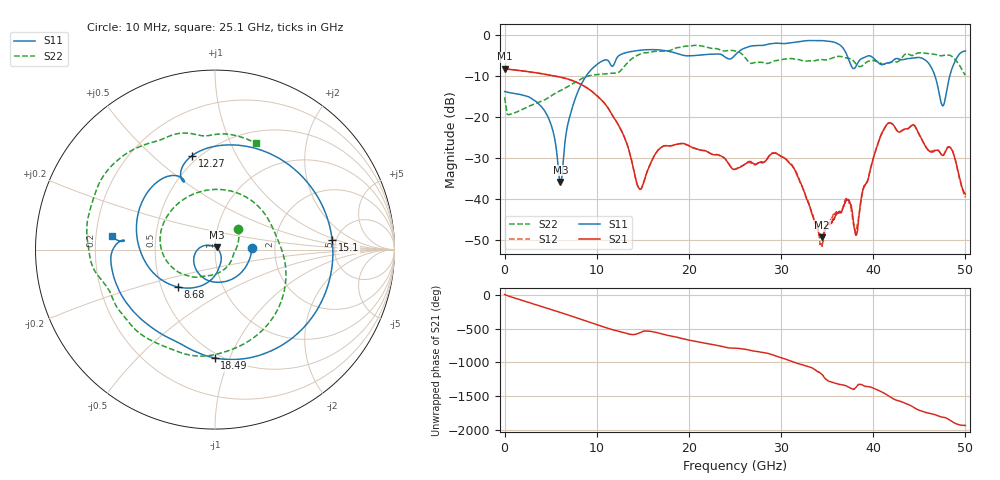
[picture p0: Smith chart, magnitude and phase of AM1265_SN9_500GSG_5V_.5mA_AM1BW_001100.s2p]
!Keysight Technologies,N5245B,MY58422270,A.16.20.02
!Date: Thursday, March 05, 2026 00:39:02
!Correction: S11(C  2-Port  )
!S21(C  2-Port  )
!S12(C  2-Port  )
!S22(C  2-Port  )
!S2P File: Measurements: S11, S21, S12, S22:
# Hz S  dB  R 50
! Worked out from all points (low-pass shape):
!   3201 points, 10 MHz to 50 GHz, reference 50 ohm
!   highest |S21| = -8.27 dB at 10 MHz (marker M1); lowest = -49.3 dB at 34.44 GHz (marker M2)
!   |S21| within 3 dB of the highest: start of sweep to 7.521 GHz
!   lowest |S11| = -35.8 dB at 6.071 GHz (marker M3), VSWR 1.03, Z = 50.9 + j1.37 ohm
!   |S11| at or under -10 dB: start of sweep to 8.867 GHz; 46.7 GHz to 48.3 GHz (1.608 GHz wide, 3.39 % of centre)
!   |S22| runs from -19.4 to -2.6 dB; largest |S21 - S12| = 0.0041
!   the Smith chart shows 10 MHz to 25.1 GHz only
!   S11 on the Smith chart (normalised r, x): 10 MHz: 1.51, +0.02; 8.68 GHz: 0.61, -0.28; 12.27 GHz: 0.46, +0.68; 15.1 GHz: 4.64, +0.85; 18.49 GHz: 0.46, -0.88; 25.1 GHz: 0.27, +0.06
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1e7  -13.80 2.2  -8.27 3.7  -8.33 3.3  -15.22 41.6
2.072088e9  -14.73 -83.3  -8.81 -88.3  -8.81 -88.3  -18.01 -72.4
4.337259e9  -18.48 -164.4  -9.58 175.5  -9.58 175.5  -15.85 -113.1
6.071288e9  -35.84 56.5  -10.30 99.6  -10.30 99.6  -13.57 -135.9
8.352081e9  -11.95 -122.1  -12.13 -5.1  -12.12 -5.0  -10.69 -175.6
8.680141e9  -10.65 -134.8  -12.55 -20.3  -12.53 -20.2  -10.35 176.2
1.227317e10  -5.37 103.7  -21.62 -177.0  -21.61 -176.8  -9.24 17.7
1.510073e10  -3.67 4.6  -35.94 -178.2  -35.86 -177.7  -4.38 -104.0
1.667854e10  -3.65 -43.1  -28.04 155.9  -28.03 156.0  -4.04 -142.3
1.849068e10  -4.39 -90.2  -26.74 98.6  -26.76 98.3  -3.28 -171.3
2.167754e10  -4.84 -145.5  -28.14 6.3  -28.21 6.5  -2.84 129.7
2.5005e10  -4.95 173.5  -32.74 -68.7  -32.73 -68.0  -3.91 71.3
2.509873e10  -4.73 172.5  -32.66 -69.3  -32.63 -68.7  -3.96 69.0
2.951972e10  -2.03 95.5  -28.88 171.1  -28.88 170.0  -6.25 -19.8
3.334708e10  -1.39 35.6  -43.58 -0.4  -43.68 -4.7  -6.34 -127.9
3.444061e10  -1.40 16.5  -49.30 -100.6  -51.21 -115.9  -6.01 -151.2
3.708071e10  -4.60 -39.8  -40.26 92.1  -39.94 93.4  -5.63 158.0
3.815862e10  -7.56 -22.8  -48.71 78.4  -47.35 72.6  -7.17 139.5
4.167354e10  -6.83 -54.7  -21.49 -56.1  -21.45 -57.4  -6.83 114.3
4.511035e10  -5.57 -102.6  -24.76 86.5  -24.83 86.9  -4.36 75.1
4.770358e10  -16.66 70.9  -29.10 -12.7  -28.91 -11.1  -4.98 40.7
5e10  -3.91 -73.4  -38.78 -132.0  -39.55 -137.3  -9.81 4.3
